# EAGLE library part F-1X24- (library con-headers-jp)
FEMALE HEADER
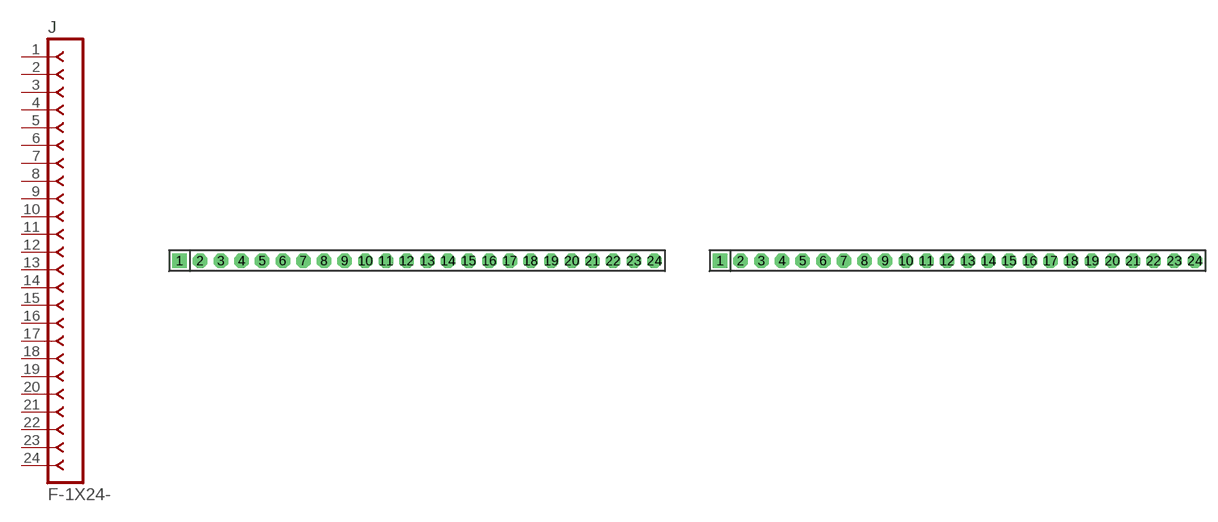
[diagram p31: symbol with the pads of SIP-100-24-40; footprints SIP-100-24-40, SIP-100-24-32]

Designator prefix J

## F-1X24-SIP-100-40  [SIP-100-24-40]
1  1  pas
2  2  pas
3  3  pas
4  4  pas
5  5  pas
6  6  pas
7  7  pas
8  8  pas
9  9  pas
10  10  pas
11  11  pas
12  12  pas
13  13  pas
14  14  pas
15  15  pas
16  16  pas
17  17  pas
18  18  pas
19  19  pas
20  20  pas
21  21  pas
22  22  pas
23  23  pas
24  24  pas

## F-1X24-SIP-100-32  [SIP-100-24-32]
Pads as for SIP-100-24-40

## F-1X24-SIP-100-32Y  [SIP-100-24-32Y]
Pads as for SIP-100-24-40

## F-1X24-SIP-100-40Y  [SIP-100-24-40Y]
Pads as for SIP-100-24-40

## F-1X24-KK-4455-B24  [KK-4455-B24]
Pads as for SIP-100-24-40

## F-1X24-KK-4455-C24  [KK-4455-C24]
Pads as for SIP-100-24-40

## F-1X24-KK-4455-A24  [KK-4455-A24]
Pads as for SIP-100-24-40

## Footprint SIP-100-24-40 (pad centres in mm)
SIP Header - 0.1", 40 mil drill
drill 1.016 pad 1.778 square: 1 -29.21,0
drill 1.016 pad 1.778 octagon: 2 -26.67,0; 3 -24.13,0; 4 -21.59,0; 5 -19.05,0; 6 -16.51,0; 7 -13.97,0; 8 -11.43,0; 9 -8.89,0; 10 -6.35,0; 11 -3.81,0; 12 -1.27,0; 13 1.27,0; 14 3.81,0; 15 6.35,0; 16 8.89,0; 17 11.43,0; 18 13.97,0; 19 16.51,0; 20 19.05,0; 21 21.59,0; 22 24.13,0; 23 26.67,0; 24 29.21,0

## Footprint SIP-100-24-32 (pad centres in mm)
SIP Header - 0.1", 32 mil drill
drill 0.813 pad 1.778 square: 1 -29.21,0
drill 0.813 pad 1.778 octagon: 2 -26.67,0; 3 -24.13,0; 4 -21.59,0; 5 -19.05,0; 6 -16.51,0; 7 -13.97,0; 8 -11.43,0; 9 -8.89,0; 10 -6.35,0; 11 -3.81,0; 12 -1.27,0; 13 1.27,0; 14 3.81,0; 15 6.35,0; 16 8.89,0; 17 11.43,0; 18 13.97,0; 19 16.51,0; 20 19.05,0; 21 21.59,0; 22 24.13,0; 23 26.67,0; 24 29.21,0

## Footprint SIP-100-24-32Y (pad centres in mm)
SIP Header - 0.1", 32 mil drill
drill 0.813 long: 1 -29.21,0; 2 -26.67,0; 3 -24.13,0; 4 -21.59,0; 5 -19.05,0; 6 -16.51,0; 7 -13.97,0; 8 -11.43,0; 9 -8.89,0; 10 -6.35,0; 11 -3.81,0; 12 -1.27,0; 13 1.27,0; 14 3.81,0; 15 6.35,0; 16 8.89,0; 17 11.43,0; 18 13.97,0; 19 16.51,0; 20 19.05,0; 21 21.59,0; 22 24.13,0; 23 26.67,0; 24 29.21,0

## Footprint SIP-100-24-40Y (pad centres in mm)
SIP Header - 0.1", 40 mil drill
drill 1.016 long: 1 -29.21,0; 2 -26.67,0; 3 -24.13,0; 4 -21.59,0; 5 -19.05,0; 6 -16.51,0; 7 -13.97,0; 8 -11.43,0; 9 -8.89,0; 10 -6.35,0; 11 -3.81,0; 12 -1.27,0; 13 1.27,0; 14 3.81,0; 15 6.35,0; 16 8.89,0; 17 11.43,0; 18 13.97,0; 19 16.51,0; 20 19.05,0; 21 21.59,0; 22 24.13,0; 23 26.67,0; 24 29.21,0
